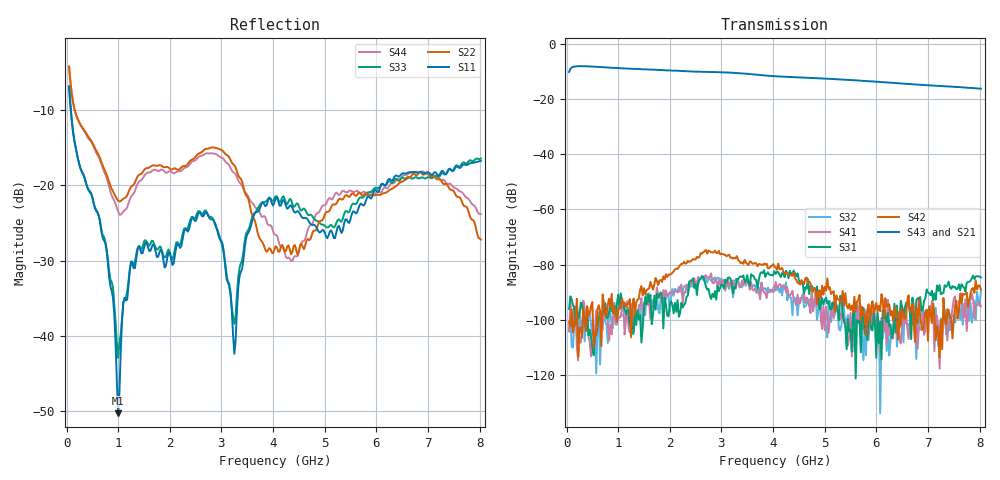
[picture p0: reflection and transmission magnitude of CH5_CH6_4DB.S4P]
!Agilent Technologies,E5071C,MY46316741,A.11.02
!Date: Mon Jun 01 10:40:40 2026
!Data & Calibration Information:
!1:CH5 INPUT 2:CH5 OUTPUT 3:CH6 INPUT 4:CH6 OUTPUT
!Freq	S11:SOLT4(ON)	S12:SOLT4(ON)	S13:SOLT4(ON)	S14:SOLT4(ON)
!	S21:SOLT4(ON)	S22:SOLT4(ON)	S23:SOLT4(ON)	S24:SOLT4(ON)
!	S31:SOLT4(ON)	S32:SOLT4(ON)	S33:SOLT4(ON)	S34:SOLT4(ON)
!	S41:SOLT4(ON)	S42:SOLT4(ON)	S43:SOLT4(ON)	S44:SOLT4(ON)
!PortZ  Port1:50+j0  Port2:50+j0  Port3:50+j0  Port4:50+j0
!Above PortZ is port z conversion or system Z0 setting when saving the data.
!When reading, reference impedance value at option line is always used.
# Hz S dB R 50
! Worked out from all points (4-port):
!   320 points, 50 MHz to 8.025 GHz, reference 50 ohm
!   strongest paths, dB at 50 MHz, 2.05 GHz, 4.05 GHz, 6.05 GHz, 8.025 GHz:
!     S43: -10.2, -9.7, -11.8, -13.8, -16.3
!     S21: -10.3, -9.9, -12.0, -14.1, -16.6
!     S42: -100.8, -83.0, -81.1, -94.8, -89.0
!     S31: -96.0, -94.6, -83.3, -108.4, -84.6
!     S41: -104.2, -90.6, -86.1, -101.6, -95.1
!     S32: -104.0, -88.7, -89.2, -100.7, -89.7
!   lowest |S11| = -50.4 dB at 1 GHz (marker M1), VSWR 1.01, Z = 49.8 - j0.199 ohm
!   |S11| at or under -10 dB: 83.27 MHz to end of sweep
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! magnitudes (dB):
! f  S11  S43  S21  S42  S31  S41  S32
! 50 MHz  -6.9  -10.2  -10.3  -100.8  -96.0  -104.2  -104.0
! 1 GHz  -50.4  -8.8  -9.0  -96.9  -90.7  -99.0  -98.4
! 1.4 GHz  -28.1  -9.2  -9.4  -92.3  -99.8  -94.6  -99.0
! 2.85 GHz  -24.7  -10.3  -10.5  -75.6  -91.7  -86.7  -85.3
! 3.25 GHz  -42.4  -10.6  -10.8  -77.5  -88.0  -87.6  -86.2
! 3.8 GHz  -22.2  -11.4  -11.6  -80.0  -83.1  -88.8  -89.5
! 8.025 GHz  -16.7  -16.3  -16.6  -89.0  -84.6  -95.1  -89.7
